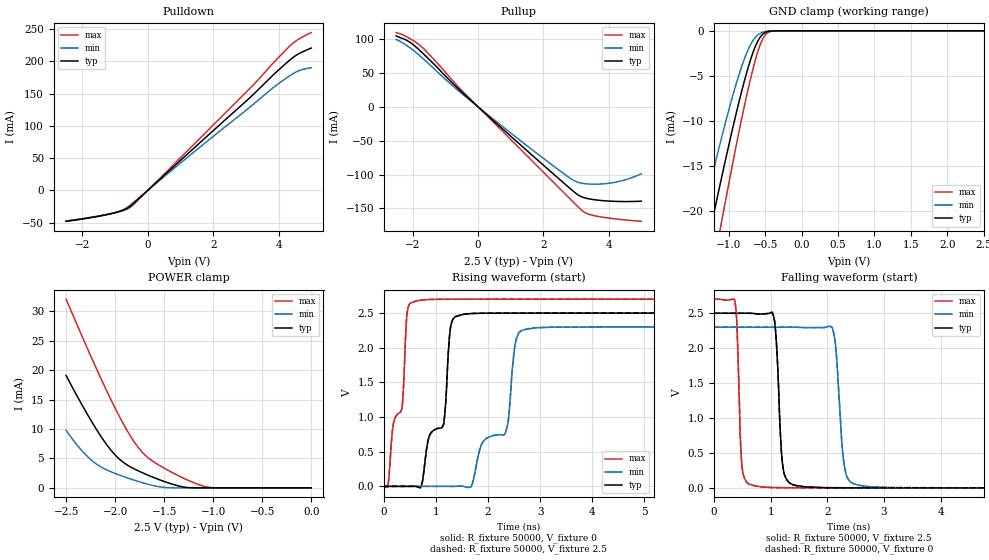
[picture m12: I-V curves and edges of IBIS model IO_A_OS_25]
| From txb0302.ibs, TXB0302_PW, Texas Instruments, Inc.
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[Model]   IO_A_OS_25
Model_type  3-state
Enable   Active-High
Vref =   0
Rref =   50000
Cref =   15p
Vmeas =   1.25
| variable   typ   min   max
C_comp   3.26pF   3.04pF   3.42pF
| C_pullup   0.87pF   0.62pF   1.16pF
| C_pulldown   0.74pF   0.58pF   0.90pF
| C_tri-state   3.26pF   3.04pF   3.42pF
[Temperature Range]   40   100   -40
| Ambient temperature   25   85   -40
[Voltage range]   2.5   2.3   2.7
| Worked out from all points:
|   slope of the pulldown table from 0 to 0.375 V, typ, clamps not added: 21.5 ohm
|   slope of the pullup table from 0 to 0.375 V, typ, clamps not added: 23 ohm
|   GND clamp passes 1 mA (typ) near -0.59 V on its own axis
|   POWER clamp passes 1 mA (typ) near -1.49 V on its own axis
|   rising waveform, R_fixture 50000, V_fixture 0: 20-80 % time 431ps typ, 669ps min, 281ps max; typ from 0 V to 2.5 V
|   falling waveform, R_fixture 50000, V_fixture 2.5: 20-80 % time 84.2ps typ, 111ps min, 62.1ps max; typ from 2.5 V to 0.001 V
|   rising waveform, R_fixture 50000, V_fixture 2.5: 20-80 % time 431ps typ, 669ps min, 281ps max; typ from 0.001 V to 2.5 V
|   falling waveform, R_fixture 50000, V_fixture 0: 20-80 % time 84.2ps typ, 111ps min, 62.1ps max; typ from 2.5 V to 0 V
[GND Clamp]
| IO_A_25
|   Voltage   I(typ)   I(min)   I(max)
-2.5V     -73.32mA   -63.17mA   -85.42mA
-1.405V   -28.12mA   -22.26mA   -34.82mA
-1.37V    -26.74mA   -21.03mA   -33.25mA
-1.23V    -21.32mA   -16.24mA   -27.03mA
-1.11V    -16.79mA   -12.29mA   -21.77mA
-940mV    -10.66mA   -7.1mA     -14.54mA
-790mV    -5.749mA   -3.248mA   -8.575mA
-665mV    -2.391mA   -1.068mA   -4.201mA
-565mV    -678.3uA   -271.2uA   -1.498mA
-490mV    -156.8uA   -67.87uA   -382.1uA
-385mV    -10.8uA    -5.431uA   -18.51uA
2.5V      503.5pA    182.5nA    46.46pA
[POWER Clamp]
| IO_A_25
|   Voltage   I(typ)   I(min)   I(max)
-2.5V     19.09mA    9.777mA    32.05mA
-2.375V   15.21mA    7.012mA    27.2mA
-2.265V   11.98mA    5.048mA    23.01mA
-2.16V    9.134mA    3.71mA     19.13mA
-2.035V   6.25mA     2.679mA    14.73mA
-1.935V   4.576mA    2.042mA    11.46mA
-1.82V    3.346mA    1.386mA    8.173mA
-1.735V   2.666mA    944.4uA    6.274mA
-1.65V    2.054mA    551.9uA    4.94mA
-1.325V   220uA      589.8nA    1.823mA
-1.05V    66.45nA    29.78nA    108uA
0V        0A         0A         0A
[Pulldown]
| IO_A_25
|   Voltage   I(typ)   I(min)   I(max)
-2.5V     -48mA      -47.93mA   -47.55mA
-1.665V   -41.59mA   -41.66mA   -41.05mA
-1.085V   -35.73mA   -35.62mA   -35.62mA
-760mV    -30.86mA   -30.01mA   -31.49mA
-515mV    -23.78mA   -21.87mA   -25.55mA
1.37V     63.57mA    57.68mA    69.48mA
3.205V    147.6mA    132.5mA    162.4mA
3.91V     182.4mA    162.1mA    201.3mA
4.47V     207mA      181.7mA    229.3mA
4.715V    214.3mA    187.1mA    237.4mA
5V        220.6mA    190.1mA    244.7mA
[Pullup]
| IO_A_25
|   Voltage   I(typ)   I(min)   I(max)
-2.5V     104.4mA    99.25mA    109.4mA
-2.08V    95.02mA    86.93mA    100.4mA
-1.69V    78.99mA    71.44mA    87.01mA
-725mV    32.23mA    28.85mA    35.93mA
25mV      -1.088mA   -975.2uA   -1.209mA
1.785V    -76.9mA    -68.1mA    -86.08mA
2.925V    -124.9mA   -108.5mA   -140.9mA
3.22V     -133.6mA   -113.1mA   -154.4mA
3.45V     -136.3mA   -114.1mA   -159.4mA
3.85V     -138.6mA   -113.7mA   -163.2mA
4.24V     -139.6mA   -111mA     -165.6mA
5V        -139.3mA   -98.95mA   -168.9mA
[Ramp]
| IO_A_25
| variable   typ   min   max
dV/dt_r   1.51/4.35E-10   1.39/6.75E-10   1.63/2.83E-10
dV/dt_f   1.51/8.82E-11   1.39/1.23E-10   1.62/6.62E-11
R_load = 50000
[Rising Waveform]
| IO_A_25
R_fixture =   50000
C_fixture =   0
L_fixture =   0
V_fixture =   0
V_fixture_min = 0
V_fixture_max = 0
|   Time   V(typ)   V(min)   V(max)
0s        2.046nV    8.984nV    417pV
349ps     55.48uV    26.05nV    1.141V
461ps     -192.9uV   208.1nV    2.572V
741ps     78.45mV    -2.709uV   2.688V
1.149ns   910.8mV    47.06uV    2.697V
1.301ns   2.366V     -137.4uV   2.698V
1.613ns   2.488V     -16.76mV   2.698V
2.573ns   2.498V     2.188V     2.699V
2.909ns   2.498V     2.287V     2.699V
37.36ns   2.499V     2.299V     2.699V
[Falling Waveform]
| IO_A_25
R_fixture =   50000
C_fixture =   0
L_fixture =   0
V_fixture =   2.5
V_fixture_min = 2.3
V_fixture_max = 2.7
|   Time   V(typ)   V(min)   V(max)
0s        2.5V       2.3V       2.7V
365ps     2.5V       2.3V       2.684V
501ps     2.5V       2.3V       254.8mV
869ps     2.49V      2.3V       12.16mV
1.069ns   2.386V     2.3V       4.783mV
1.237ns   205.7mV    2.3V       2.796mV
1.613ns   14.14mV    2.294V     1.519mV
2.085ns   2.54mV     2.297V     1.224mV
2.765ns   1.32mV     14.69mV    1.137mV
37.36ns   1.071mV    1.083mV    1.062mV
[Rising Waveform]
| IO_A_25
R_fixture =   50000
C_fixture =   0
L_fixture =   0
V_fixture =   2.5
V_fixture_min = 2.3
V_fixture_max = 2.7
|   Time   V(typ)   V(min)   V(max)
0s        1.07mV     1.078mV    1.062mV
349ps     1.126mV    1.078mV    1.142V
461ps     877.2uV    1.078mV    2.573V
741ps     79.52mV    1.075mV    2.689V
1.149ns   912mV      1.125mV    2.698V
1.301ns   2.367V     939.9uV    2.699V
1.613ns   2.49V      -15.69mV   2.7V
2.325ns   2.499V     762.1mV    2.7V
2.901ns   2.5V       2.288V     2.7V
37.36ns   2.5V       2.3V       2.7V
[Falling Waveform]
| IO_A_25
R_fixture =   50000
C_fixture =   0
L_fixture =   0
V_fixture =   0
V_fixture_min = 0
V_fixture_max = 0
|   Time   V(typ)   V(min)   V(max)
0s        2.499V     2.299V     2.699V
365ps     2.499V     2.299V     2.683V
501ps     2.499V     2.299V     253.6mV
869ps     2.489V     2.299V     11.1mV
1.069ns   2.385V     2.299V     3.721mV
1.237ns   204.6mV    2.299V     1.735mV
1.613ns   13.07mV    2.293V     457.7uV
2.085ns   1.47mV     2.296V     162.4uV
2.765ns   249.9uV    13.6mV     75.55uV
37.36ns   1.195uV    5.131uV    451.5nV
